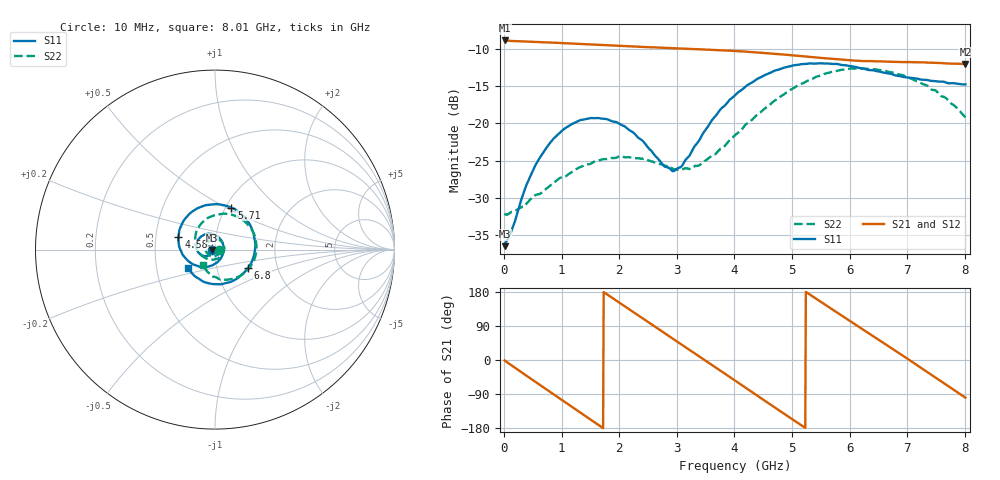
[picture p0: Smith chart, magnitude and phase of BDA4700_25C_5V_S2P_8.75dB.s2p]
!Agilent Technologies,E5071B,MY42404982,A.09.10
!Date: Mon Oct 20 13:30:23 2025
!Data & Calibration Information:
!Freq	S11:SOLT2(ON)	S21:SOLT2(ON)	S12:SOLT2(ON)	S22:SOLT2(ON)
# Hz S RI R 50
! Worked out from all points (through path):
!   801 points, 10 MHz to 8.01 GHz, reference 50 ohm
!   highest |S21| = -8.87 dB at 20 MHz (marker M1); lowest = -12.0 dB at 8.01 GHz (marker M2)
!   group delay of S21, straight-line fit = 283 ps
!   lowest |S11| = -36.5 dB at 10 MHz (marker M3), VSWR 1.03, Z = 48.5 - j0.146 ohm
!   |S11| at or under -10 dB: start of sweep to end of sweep
!   |S22| runs from -32.3 to -12.6 dB; largest |S21 - S12| = 0.0027
!   S11 on the Smith chart (normalised r, x): 10 MHz: 0.97, -0.00; 4.58 GHz: 0.66, +0.09; 5.71 GHz: 1.06, +0.53; 6.8 GHz: 1.41, -0.30; 8.01 GHz: 0.73, -0.16
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1e7  -0.0149 -0.00151  0.36 -0.00787  0.3601 -0.00811  0.0248 -0.0013
2e7  -0.0155 -0.00235  0.3599 -0.0139  0.3599 -0.0152  0.0245 -0.00136
4.1e8  -0.0282 -0.0287  0.2565 -0.2437  0.2564 -0.2439  0.0187 -0.0227
7.2e8  -0.0563 -0.0365  0.0848 -0.3394  0.0847 -0.3393  -0.000163 -0.0361
1.02e9  -0.0875 -0.0217  -0.1023 -0.3303  -0.1025 -0.3307  -0.0274 -0.0339
1.35e9  -0.1044 0.0169  -0.2672 -0.2125  -0.2673 -0.2127  -0.0509 -0.0069
1.93e9  -0.0585 0.084  -0.3097 0.1216  -0.3099 0.1218  -0.0251 0.0529
2.32e9  0.00112 0.0808  -0.1564 0.2874  -0.1563 0.2874  0.0218 0.0542
2.68e9  0.0418 0.0394  0.0462 0.3194  0.046 0.3194  0.0498 0.0194
2.96e9  0.0471 -0.0101  0.1909 0.2554  0.1911 0.2552  0.047 -0.0143
3.37e9  0.00621 -0.0748  0.3082 0.062  0.3086 0.0618  0.0104 -0.0509
3.68e9  -0.0585 -0.0967  0.291 -0.1078  0.291 -0.1088  -0.0324 -0.0537
4.01e9  -0.1358 -0.0737  0.179 -0.2486  0.1791 -0.2483  -0.0769 -0.0313
4.58e9  -0.2036 0.0687  -0.1149 -0.2722  -0.1148 -0.2724  -0.1098 0.0696
4.98e9  -0.1529 0.1882  -0.2569 -0.1267  -0.2575 -0.1273  -0.068 0.1542
5.35e9  -0.0406 0.2489  -0.273 0.0549  -0.2733 0.0542  0.0242 0.1966
5.71e9  0.0906 0.2338  -0.183 0.1999  -0.1827 0.2  0.1301 0.1807
6.18e9  0.2069 0.1112  0.0198 0.2616  0.0215 0.2622  0.2231 0.0682
6.68e9  0.2059 -0.0652  0.2102 0.1517  0.2109 0.1513  0.2073 -0.0784
6.8e9  0.1834 -0.102  0.2364 0.1042  0.2371 0.1033  0.1882 -0.1063
7.32e9  0.0357 -0.1929  0.2247 -0.1232  0.2244 -0.124  0.066 -0.1687
8.01e9  -0.1495 -0.1048  -0.0408 -0.2471  -0.0405 -0.2475  -0.065 -0.0883
